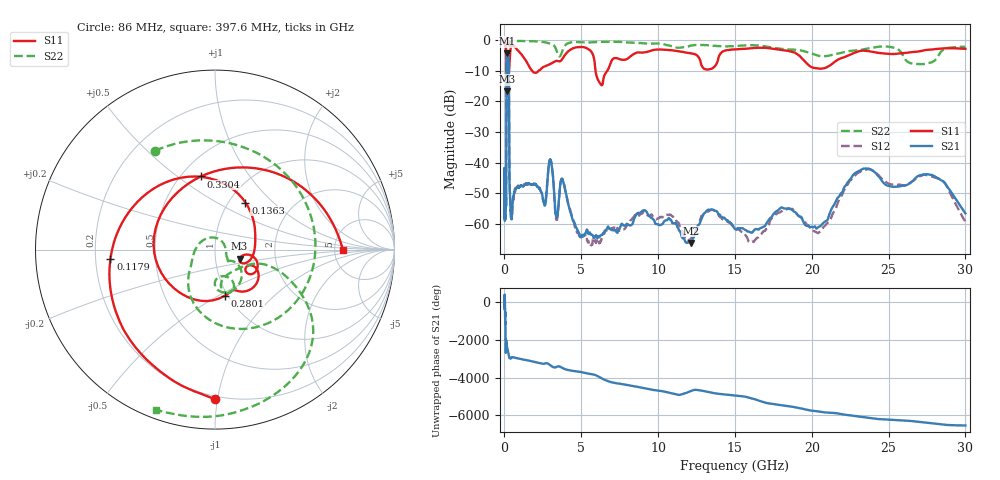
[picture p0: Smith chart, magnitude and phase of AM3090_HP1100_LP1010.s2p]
! Date/Time: Thu, Feb 28, 2019 2:07 PM
! Network Analyzer: Agilent Technologies E8364B Rev: A.07.50.67
! Sweep from 0.010 to 30.000 GHz, 1601 Points, Sweep Type: LOG
! Power Supply: 5.023 V, 0.002 A
# Hz S DB R 50
!freq MagS11 AngS11 MagS21 AngS21 MagS12 AngS12 MagS22 AngS22
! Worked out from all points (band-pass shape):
!   1601 points, 10 MHz to 30 GHz, reference 50 ohm
!   highest |S21| = -4.32 dB at 191.5 MHz (marker M1); lowest = -66.2 dB at 12.13 GHz (marker M2)
!   |S21| within 3 dB of the highest: 142.8 MHz to 274.8 MHz (131.9 MHz wide, 63.2 % of centre)
!   lowest |S11| = -16.7 dB at 167.3 MHz (marker M3), VSWR 1.34, Z = 65.4 - j6.84 ohm
!   |S11| at or under -10 dB: 136 MHz to 301.2 MHz (165.2 MHz wide, 75.5 % of centre); 1.791 GHz to 2.23 GHz (439.5 MHz wide, 21.9 % of centre); 5.926 GHz to 6.699 GHz (773.2 MHz wide, 12.2 % of centre)
!   |S22| runs from -24.7 to -0.2 dB; largest |S21 - S12| = 0.014
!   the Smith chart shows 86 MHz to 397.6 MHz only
!   S11 on the Smith chart (normalised r, x): 86 MHz: 0.18, -0.98; 117.9 MHz: 0.26, -0.04; 136.3 MHz: 1.19, +0.69; 280.1 MHz: 0.97, -0.54; 330.4 MHz: 0.62, +0.61; 397.6 MHz: 5.97, -0.11
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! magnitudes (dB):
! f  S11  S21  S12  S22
! 10 MHz  -0.3  -42.1  -41.4  -0.7
! 38.04 MHz  -0.4  -57.1  -56.9  -1.4
! 86 MHz  -1.6  -53.1  -53.8  -3.8
! 117.9 MHz  -4.7  -38.2  -37.9  -5.2
! 136.3 MHz  -10.1  -11.0  -11.0  -18.8
! 144.7 MHz  -12.8  -6.8  -6.7  -24.6
! 167.3 MHz  -16.7  -4.6  -4.5  -18.4
! 191.5 MHz  -11.9  -4.3  -4.3  -12.1
! 280.1 MHz  -11.6  -8.4  -8.4  -14.5
! 330.4 MHz  -7.6  -46.5  -46.4  -1.1
! 397.6 MHz  -2.9  -55.7  -55.4  -0.4
! 550.5 MHz  -1.9  -52.5  -52.5  -0.3
! 2.084 GHz  -10.7  -47.3  -47.5  -0.5
! 2.987 GHz  -7.8  -39.0  -38.9  -1.2
! 3.385 GHz  -6.8  -58.0  -58.6  -3.4
! 3.76 GHz  -6.2  -45.3  -45.3  -3.7
! 5.501 GHz  -3.1  -63.3  -66.9  -0.8
! 7.926 GHz  -6.3  -60.1  -60.9  -0.8
! 12.13 GHz  -4.4  -66.2  -65.1  -1.8
! 20.41 GHz  -9.3  -61.1  -63.0  -5.1
! 23.48 GHz  -3.5  -41.9  -42.3  -2.9
! 30 GHz  -2.9  -56.6  -59.3  -2.2
